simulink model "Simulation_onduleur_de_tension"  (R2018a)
settings: Solver=FixedStepAuto  StartTime=0.0  StopTime=0.1  MaxStep=Ts  RelTol=1e-3
PreLoadFcn:
  | Ts=1/60/3240;
InitFcn:
  | Ts=1/60/3240;
libraries: powerlib x10, powerlib_meascontrol x1

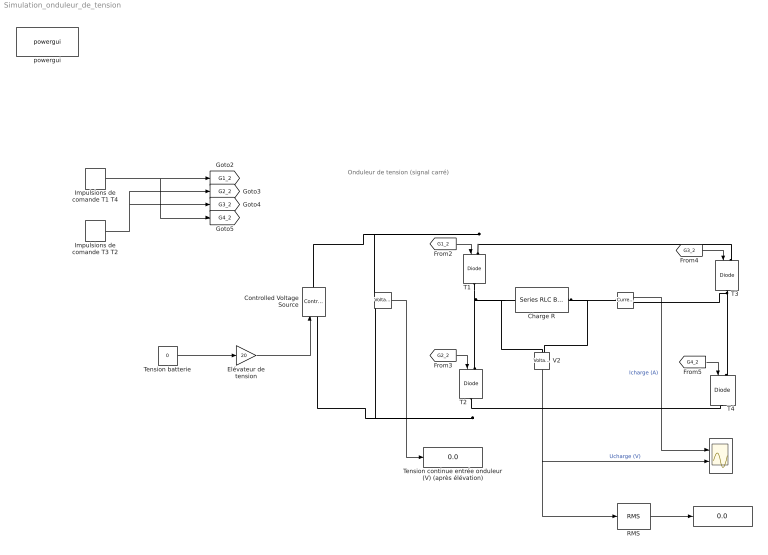
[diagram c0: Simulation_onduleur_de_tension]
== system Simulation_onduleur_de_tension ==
  note: Onduleur de tension (signal carré)
  " " : powerlib/Measurements/Voltage Measurement  Tag=PoWeRsYsTeMmEaSuReMeNt  PhasorSimulation=off  OutputType=Magnitude  PSBequivalent=0
  "    " : powerlib/Measurements/Current Measurement  PhasorSimulation=off  OutputType=Complex  PSBequivalent=0
  "     " : Scope  NumInputPorts=2
  "      " : Display
  Charge R : powerlib/Elements/Series RLC Branch  LConnTagsString=__new0  RConnTagsString=__new0  BranchType=R  Resistance=240  Inductance=1e-2  SetiL0=off  InitialCurrent=0  Capacitance=100e-3  Setx0=off  InitialVoltage=0  Measurements=Branch voltage and current
  Controlled Voltage Source : powerlib/Electrical Sources/Controlled Voltage Source  Initialize=on  Source_Type=DC  Amplitude=0  Phase=0  Frequency=0  Measurements=None
  Elévateur de tension : Gain  Gain=20
  Impulsions de comande T1 T4 : DiscretePulseGenerator  PulseType=Time based  Period=0.02  PulseWidth=50
  Impulsions de comande T3 T2 : DiscretePulseGenerator  PulseType=Time based  Period=0.02  PulseWidth=50  PhaseDelay=0.01
  RMS : powerlib_meascontrol/Measurements/RMS  TrueRMS=on  Freq=60  RMSInit=120  Ts=0
  T{1..4} (4 alike) : powerlib/Power Electronics/IGBT//Diode  Ron=1e-3  Rs=1e5  Cs=inf  Measurements=off
  Tension batterie : Constant  Value=0
  Tension continue entrée onduleur (V) (après élévation) : Display
  V2 : powerlib/Measurements/Voltage Measurement  Tag=PoWeRsYsTeMmEaSuReMeNt  PhasorSimulation=off  OutputType=Magnitude  PSBequivalent=0
  powergui : powerlib/powergui  SimulationMode=Discrete  SampleTime=Ts  frequency=60  Iterations=50  frequencyindice=0  Pbase=100e6  ErrMax=1e-4  UnitsV=kV  UnitsW=MW  buscounter=0  FunctionMessages=off  echomessages=off  EnableUseOfTLC=off  CurrentSourceSwitches=off  DisableSnubberDevices=off  DisableRonSwitches=off  DisableVfSwitches=off  DisplayEquations=off  SolverType=Tustin/Backward Euler (TBE)  Interpol=off  ExternalGateDelay=off  methode=off  Ts=100  x0status=blocks  SPID=off  SwTol=0  HookPort=off  RestoreLinks=warning  ResistiveCurrentMeasurement=off  Frange=[0:2:500]  Ylog=off  Xlog=on  ShowGrid=off  save=off  variable=ZData  structure=sps1phPWM1_str  ZoomFFT=on  StartTime=0.1-2/60  cycles=2  DisplayStyle=1  fundamental=60  FreqAxis=off  MaxFrequency=5000  frequencyindicesteady=1  RmsSteady=1  display=off
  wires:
  [G1_2] -> T1/1
  [G2_2] -> T2/1
  [G3_2] -> T3/1
  [G4_2] -> T4/1
  Impulsions de comande T1 T4/1 -> [G4_2], [G1_2]
  Impulsions de comande T3 T2/1 -> [G3_2], [G2_2]
  V2/1 -> RMS/1, "     "/2  "Ucharge (V)"
  Tension batterie/1 -> Elévateur de tension/1
  Elévateur de tension/1 -> Controlled Voltage Source/1
  " "/1 -> Tension continue entrée onduleur (V) (après élévation)/1
  RMS/1 -> "      "/1
  "    "/1 -> "     "/1  "Icharge (A)"
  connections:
  T2/RConn1 -- " "/LConn2 -- Controlled Voltage Source/LConn1 -- T4/RConn1
  T3/LConn1 -- Controlled Voltage Source/RConn1 -- " "/LConn1 -- T1/LConn1
  T1/RConn1 -- V2/LConn1 -- Charge R/LConn1 -- T2/LConn1
  Charge R/RConn1 -- V2/LConn2 -- "    "/LConn1
  T3/RConn1 -- "    "/RConn1 -- T4/LConn1
